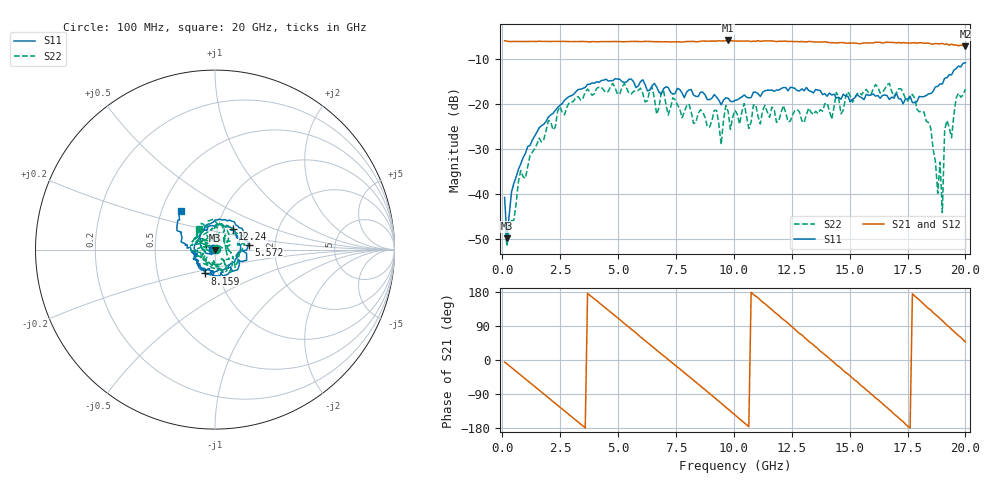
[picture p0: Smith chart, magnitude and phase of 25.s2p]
!Agilent Technologies,N5230C,MY49001569,A.09.33.09
!Agilent N5230C: A.09.33.09
!Date: Monday, July 20, 2015 16:56:43
!Correction: S11(Full 2 Port(1,2))
!S21(Full 2 Port(1,2))
!S12(Full 2 Port(1,2))
!S22(Full 2 Port(1,2))
!S2P File: Measurements: S11, S21, S12, S22:
# Hz S  dB  R 50
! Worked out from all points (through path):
!   201 points, 100 MHz to 20 GHz, reference 50 ohm
!   highest |S21| = -5.90 dB at 9.752 GHz (marker M1); lowest = -7.2 dB at 20 GHz (marker M2)
!   group delay of S21, straight-line fit = 143 ps
!   lowest |S11| = -49.8 dB at 199.5 MHz (marker M3), VSWR 1.01, Z = 50 - j0.323 ohm
!   |S11| at or under -10 dB: start of sweep to end of sweep
!   |S22| runs from -51.5 to -15.4 dB; largest |S21 - S12| = 0.015
!   S11 on the Smith chart (normalised r, x): 100 MHz: 0.98, +0.00; 5.572 GHz: 1.46, +0.08; 8.159 GHz: 0.86, -0.23; 12.24 GHz: 1.18, +0.28; 20 GHz: 0.63, +0.29
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1e8  -40.71 173.2  -5.97 -5.6  -6.04 -5.2  -46.28 27.5
1.995e8  -49.79 -94.7  -6.05 -10.0  -6.13 -10.2  -51.52 -33.7
3.985e8  -39.49 -83.8  -6.15 -20.0  -6.16 -20.1  -45.86 -79.5
1.095e9  -29.44 -126.0  -6.12 -54.8  -6.12 -54.6  -33.97 -139.2
3.483e9  -16.53 97.6  -6.12 -174.0  -6.14 -174.4  -18.70 93.8
5.5725e9  -14.47 8.4  -6.09 81.3  -6.15 81.1  -17.77 -16.8
6.7665e9  -17.37 -49.8  -6.17 20.8  -6.16 20.7  -20.79 -54.8
8.1595e9  -16.78 -113.2  -6.12 -48.2  -6.12 -48.8  -21.77 -144.8
9.254e9  -18.45 -164.5  -6.04 -104.1  -5.94 -104.3  -21.39 154.4
9.453e9  -20.17 -176.4  -6.01 -113.9  -6.03 -114.3  -28.95 139.7
9.7515e9  -18.73 164.9  -5.90 -129.7  -6.02 -130.2  -21.59 143.3
1.005e10  -19.19 147.6  -6.02 -145.4  -6.01 -145.4  -21.41 106.9
1.2239e10  -16.35 49.5  -6.04 102.4  -6.11 101.2  -21.92 -44.7
1.3433e10  -17.54 11.6  -6.19 40.1  -6.31 39.5  -22.36 -131.6
1.5224e10  -18.62 -81.0  -6.49 -53.2  -6.51 -52.6  -18.66 139.8
1.67165e10  -18.98 -150.1  -6.33 -131.4  -6.18 -131.5  -15.43 93.8
1.8408e10  -17.73 -174.5  -6.48 135.6  -6.56 136.4  -24.12 3.2
1.8806e10  -16.10 170.3  -6.62 114.8  -6.56 113.9  -39.79 29.1
1.89055e10  -15.54 171.7  -6.67 109.5  -6.59 108.3  -32.89 -28.5
1.9005e10  -15.54 169.2  -6.55 103.7  -6.54 103.0  -44.07 -49.0
1.91045e10  -14.27 167.2  -6.76 98.0  -6.62 97.0  -25.74 158.0
2e10  -10.84 131.7  -7.20 47.6  -7.14 47.5  -16.69 128.7
